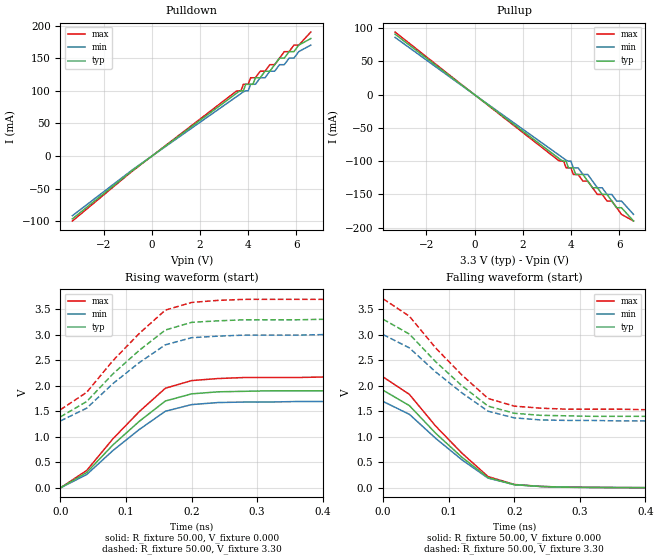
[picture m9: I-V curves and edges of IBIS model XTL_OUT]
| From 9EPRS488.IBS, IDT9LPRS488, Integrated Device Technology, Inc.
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|   Model XTL_OUT
[Model]   XTL_OUT
Model_type   Output
Polarity   Non-Inverting
Enable   Active-High
Vmeas =   1.50V
Cref =   5.00pF
Rref =  0.000
Vref =   1.50V
C_comp   3.40pF   2.85pF   3.95pF
[Temperature Range]   27.00   70.00   0.000
[Voltage Range]   3.30V   3.00V   3.70V
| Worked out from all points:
|   slope of the pulldown table from 0 to 0.495 V, typ, clamps not added: 36.5 ohm
|   slope of the pullup table from 0 to 0.495 V, typ, clamps not added: 36.5 ohm
|   rising waveform, R_fixture 50.00, V_fixture 0.000: 20-80 % time 96.7ps typ, 96.9ps min, 95.3ps max; typ from 0 V to 1.91 V
|   rising waveform, R_fixture 50.00, V_fixture 3.30: 20-80 % time 96.7ps typ, 96.9ps min, 95.3ps max; typ from 1.39 V to 3.3 V
|   falling waveform, R_fixture 50.00, V_fixture 0.000: 20-80 % time 95.7ps typ, 96.1ps min, 95.3ps max; typ from 1.91 V to 0 V
|   falling waveform, R_fixture 50.00, V_fixture 3.30: 20-80 % time 96ps typ, 96.9ps min, 95.3ps max; typ from 3.3 V to 1.39 V
[Pulldown]
| voltage   I(typ)   I(min)   I(max)
-3.3V     -96.11mA   -91.26mA   -99.37mA
-700mV    -19.16mA   -18.15mA   -19.85mA
3.5V      95.79mA    90.64mA    99.24mA
3.7V      100mA      95.83mA    100mA
3.8V      100mA      98.44mA    110mA
3.9V      110mA      100mA      110mA
4.2V      110mA      110mA      120mA
4.3V      120mA      110mA      120mA
4.9V      130mA      130mA      140mA
5.1V      140mA      130mA      140mA
5.3V      150mA      140mA      150mA
6.6V      180mA      170mA      190mA
[Pullup]
| voltage   I(typ)   I(min)   I(max)
-3.3V     91.08mA    86.24mA    94.33mA
3.7V      -100mA     -95.84mA   -100mA
3.8V      -100mA     -98.55mA   -110mA
4.2V      -120mA     -110mA     -120mA
4.5V      -120mA     -120mA     -130mA
4.7V      -130mA     -120mA     -130mA
4.9V      -140mA     -130mA     -140mA
5.5V      -150mA     -150mA     -160mA
5.7V      -160mA     -150mA     -160mA
5.9V      -170mA     -160mA     -170mA
6.1V      -170mA     -160mA     -180mA
6.6V      -190mA     -180mA     -190mA
[Ramp]
| variable   typ   min   max
dV/dt_r   1.14/82.10p   1.02/83.53p   1.30/81.21p
dV/dt_f   1.14/81.65p   1.02/83.01p   1.30/80.69p
R_load = 50.00
[Rising Waveform]
R_fixture = 50.00
V_fixture = 0.000
V_fixture_min = 0.000
V_fixture_max = 0.000
| time   V(typ)   V(min)   V(max)
0s        0V         0V         0V
40ps      300mV      260mV      340mV
80ps      840mV      730mV      960mV
120ps     1.3V       1.14V      1.49V
160ps     1.7V       1.5V       1.95V
200ps     1.84V      1.63V      2.1V
240ps     1.88V      1.67V      2.14V
280ps     1.89V      1.68V      2.16V
400ps     1.9V       1.69V      2.17V
2ns       1.91V      1.69V      2.17V
[Rising Waveform]
R_fixture = 50.00
V_fixture = 3.30
V_fixture_min = 3.00
V_fixture_max = 3.70
| time   V(typ)   V(min)   V(max)
0s        1.39V      1.31V      1.53V
40ps      1.69V      1.56V      1.87V
80ps      2.23V      2.04V      2.49V
120ps     2.69V      2.45V      3.02V
160ps     3.09V      2.8V       3.48V
200ps     3.24V      2.94V      3.63V
240ps     3.27V      2.97V      3.67V
280ps     3.29V      2.99V      3.69V
440ps     3.3V       3V         3.7V
2ns       3.3V       3V         3.7V
[Falling Waveform]
R_fixture = 50.00
V_fixture = 0.000
V_fixture_min = 0.000
V_fixture_max = 0.000
| time   V(typ)   V(min)   V(max)
0s        1.91V      1.69V      2.17V
40ps      1.61V      1.44V      1.83V
80ps      1.07V      970mV      1.21V
120ps     600mV      550mV      680mV
160ps     200mV      190mV      220mV
200ps     62.62mV    61.59mV    66.41mV
240ps     26.92mV    26.77mV    28.3mV
280ps     11.8mV     12.24mV    12.41mV
400ps     3.44mV     3.46mV     3.52mV
2ns       0V         0V         0V
[Falling Waveform]
R_fixture = 50.00
V_fixture = 3.30
V_fixture_min = 3.00
V_fixture_max = 3.70
| time   V(typ)   V(min)   V(max)
0s        3.3V       3V         3.7V
40ps      3.01V      2.74V      3.36V
80ps      2.47V      2.27V      2.74V
120ps     2V         1.86V      2.21V
160ps     1.6V       1.5V       1.75V
200ps     1.46V      1.37V      1.6V
240ps     1.42V      1.33V      1.56V
280ps     1.41V      1.32V      1.54V
400ps     1.4V       1.31V      1.53V
2ns       1.39V      1.31V      1.53V
